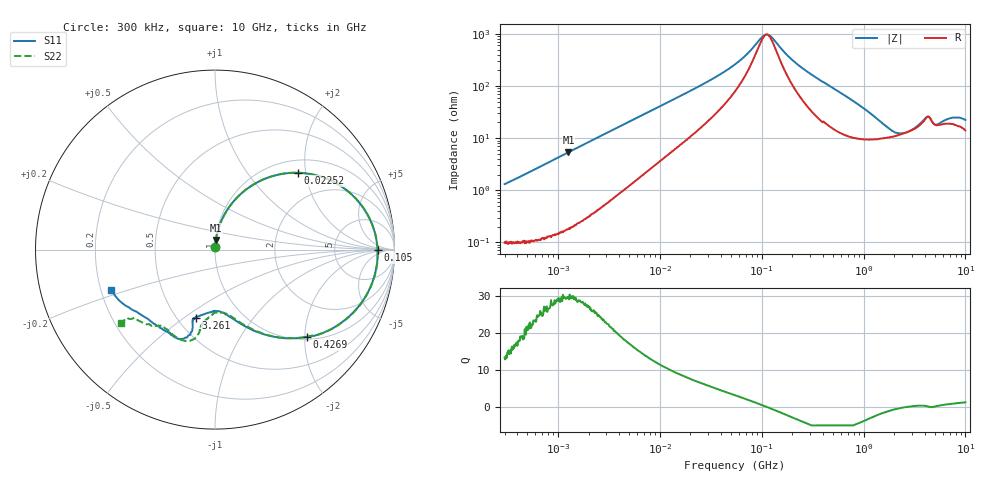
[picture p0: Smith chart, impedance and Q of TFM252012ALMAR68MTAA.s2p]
! S-Parameter Data Generated by TDK Corporation
! Copyright(C) 2019 TDK Corporation.
! All Rights Reserved.
! TDK P/N: TFM252012ALMAR68MTAA (Inductor)
! Property: L=680nH at 1MHz
! Size(LxWxT):
! Model Type: s2p (Touchstone File Format Version 1.0)
! Frequency: DC=Yes Start=0.3MHz Stop=10000MHz 802points Log-sweep
! Model Generated on Sep. 23, 2019
! Port Assignments:
!  1 ---@@@--- 2
! Applicable Conditions:
!  Temperature = 25 degC
!  DC Bias Current = 0 A
!  Small Signal Operation
! Terms and conditions regarding TDK Simulation Models
! (1)This simulation model is being provided solely for informational purposes. Please refer to the specifications of the products in terms of detailed characteristics of such products.
! (2)In no event shall TDK Corporation of any of its subsidiaries be liable for any loss or damage arising, directly or indirectly,
!  From any information contained in this simulation model, including, but not limited to loss or damages arising from any inaccuracies, omissions or errors in connection with such information.
! (3)Any and all copyrights on this simulation model are owned by TDK Corporation.
!  Duplication or redistribution of this simulation model without prior written permission from TDK Corporation is prohibited.
! (4)This simulation model is subject to any modification or change without any prior notice.
! (5)Neither TDK Corporation nor any of its subsidiaries shall make any warranty, express or implied,
!  Including but not limited to the correctness, implied warranties of merchantability and fitness for a particular purpose with respect to this simulation models.
! (6)The use of this simulation model shall be deemed to have consented to the terms and conditions hereof.
# Hz S MA R 50
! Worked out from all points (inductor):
!   801 points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, 300 kHz to 10 GHz, reference 50 ohm
!   read as one part in series: L = 682 nH near 318.3 kHz
!   highest Q = 29.5 at 1.271 MHz (marker M1), where L = 671 nH
!   self-resonance near 112.1 MHz
!   S11 on the Smith chart (normalised r, x): 300 kHz: 1.00, +0.03; 22.52 MHz: 1.28, +1.81; 105 MHz: 20, -1; 426.9 MHz: 1.06, -2.05; 3.261 GHz: 0.62, -0.55; 10 GHz: 0.24, -0.18
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300000  0.01428 86.4  0.9985 -0.7  0.9985 -0.7  0.01427 87.7
1271272  0.0535 85.2  0.9965 -3.1  0.9966 -3.1  0.05355 85.2
1713600  0.0718 83.9  0.9947 -4.1  0.9947 -4.1  0.07179 84.0
4796912  0.1924 75.6  0.9702 -11.1  0.9705 -11.1  0.1924 75.6
9671944  0.3555 64.2  0.9044 -20.9  0.9049 -20.9  0.3555 64.2
2.252362e7  0.6294 42.9  0.6921 -38.9  0.6924 -38.9  0.6296 42.9
3.424315e7  0.7528 30.7  0.5284 -48.2  0.5286 -48.2  0.7531 30.7
5.477226e7  0.8496 17.3  0.3285 -55.0  0.3286 -55.0  0.85 17.3
7.244865e7  0.8843 9.7  0.2136 -53.2  0.2136 -53.2  0.8848 9.8
1.050124e8  0.9055 -0.1  0.09781 -16.9  0.09786 -16.9  0.9064 -0.1
1.210198e8  0.9063 -4.0  0.09859 16.2  0.0986 16.2  0.9074 -3.9
2.013356e8  0.8738 -18.6  0.2777 52.5  0.2777 52.5  0.875 -18.5
3.126428e8  0.7938 -33.0  0.4742 46.1  0.4743 46.1  0.7955 -32.9
4.269249e8  0.7054 -43.6  0.6003 37.3  0.6004 37.3  0.7075 -43.3
6.076905e8  0.5866 -55.9  0.7228 25.7  0.723 25.7  0.5891 -55.5
9.101824e8  0.4563 -68.9  0.8107 11.8  0.8109 11.8  0.4603 -67.8
1.767019e9  0.3427 -87.7  0.844 -10.9  0.8442 -10.9  0.3523 -84.1
3.261479e9  0.3955 -105.8  0.7689 -34.4  0.769 -34.5  0.4112 -98.8
4.166115e9  0.4602 -105.9  0.6686 -43.9  0.669 -43.9  0.4688 -100.7
4.865898e9  0.5376 -113.3  0.6617 -44.0  0.6618 -44.0  0.5356 -112.4
7.06055e9  0.5343 -127.2  0.6191 -66.3  0.6193 -66.4  0.5442 -129.4
1e10  0.6194 -158.6  0.4928 -87.6  0.4936 -87.8  0.663 -141.8
